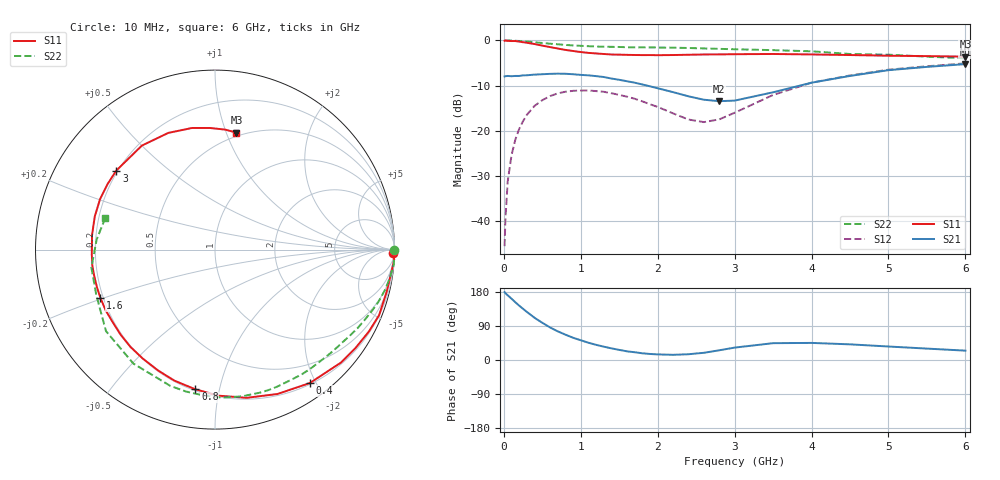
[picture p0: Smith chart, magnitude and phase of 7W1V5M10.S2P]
! Infineon Technologies  Discrete & RF Semiconductors
! BFS17W
! Si NPN RF Bipolar Junction Transistor in SOT323
! VCE = 1.5 V  IC = 0.1 mA
! Common Emitter S-Parameters:  August  1999
# GHz  S  MA  R  50
!  f  S11  S21  S12  S22
! GHz  MAG  ANG  MAG  ANG  MAG  ANG  MAG  ANG
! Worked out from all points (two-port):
!   36 points, 10 MHz to 6 GHz, reference 50 ohm
!   highest |S21| = -5.24 dB at 6 GHz (marker M1); lowest = -13.4 dB at 2.8 GHz (marker M2)
!   |S21| within 3 dB of the highest: start of sweep to 1.345 GHz; 4.37 GHz to end of sweep
!   lowest |S11| = -3.6 dB at 6 GHz (marker M3), VSWR 4.93, Z = 23.4 + j54.3 ohm
!   |S11| at or under -10 dB: nowhere
!   |S22| runs from -3.9 to 0.0 dB; largest |S21 - S12| = 0.4
!   S11 on the Smith chart (normalised r, x): 10 MHz: 27, -87; 400 MHz: 0.22, -1.92; 800 MHz: 0.21, -0.85; 1.6 GHz: 0.19, -0.20; 3 GHz: 0.19, +0.34; 6 GHz: 0.47, +1.09
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0.01  0.9936 -1.2  0.4 179.1  0.0053 86.8  0.9999 0.0
0.02  0.9999 -3.2  0.402 176.4  0.0103 87.7  0.9958 -0.9
0.05  0.9907 -7.1  0.405 170.8  0.0274 85.6  0.9983 -2.4
0.1  0.9849 -13.9  0.402 161.7  0.0539 80.2  0.9989 -4.8
0.2  0.9713 -28.0  0.405 143.3  0.1052 71.4  0.9858 -9.3
0.3  0.943 -41.8  0.412 126.8  0.1507 62.2  0.9721 -13.7
0.4  0.9122 -54.6  0.419 111.3  0.1892 53.9  0.955 -17.9
0.6  0.8445 -77.9  0.427 86.0  0.2424 39.5  0.9207 -25.3
0.8  0.786 -98.0  0.428 66.9  0.2708 27.7  0.8926 -32.2
1.1  0.7284 -123.5  0.411 45.5  0.2794 13.9  0.864 -41.9
1.3  0.7079 -138.0  0.394 35.1  0.2705 6.9  0.8521 -48.6
1.6  0.6929 -157.1  0.354 22.9  0.2387 -0.7  0.8416 -58.5
2.2  0.6898 173.3  0.268 13.7  0.1561 0.8  0.8313 -79.7
2.6  0.6995 156.3  0.221 19.0  0.1249 24.3  0.8154 -94.3
2.8  0.7011 148.6  0.213 25.6  0.1339 39.0  0.8072 -101.5
3  0.7045 141.3  0.216 32.7  0.1585 49.7  0.7992 -108.1
3.5  0.7084 125.1  0.267 44.4  0.2496 57.5  0.7811 -125.6
4  0.7003 111.8  0.341 45.1  0.3409 52.9  0.7585 -143.2
4.5  0.6896 100.7  0.405 41.3  0.4102 45.8  0.7085 -158.9
5  0.6781 92.3  0.469 35.6  0.4747 38.9  0.696 -171.7
5.5  0.671 85.2  0.51 30.1  0.5182 32.1  0.6616 175.1
6  0.6626 79.6  0.547 24.7  0.5578 26.0  0.6359 163.7
